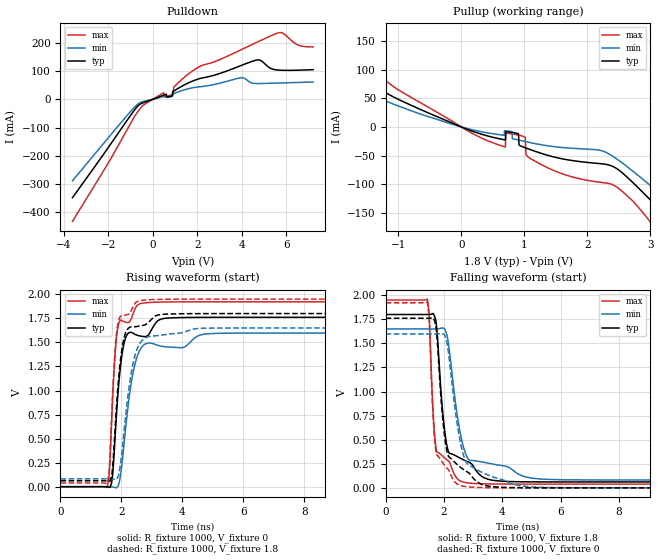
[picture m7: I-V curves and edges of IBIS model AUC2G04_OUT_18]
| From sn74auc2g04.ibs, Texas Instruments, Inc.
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[Model]   AUC2G04_OUT_18
Model_type  Output
Vref =   0
Rref =   1000
Cref =   30p
Vmeas =   0.9
| variable   typ   min   max
C_comp   6.69pF   0.47pF   21.38pF
| C_pullup   7.14pF   1.04pF   21.38pF
| C_pulldown   6.23pF   0.47pF   15.44pF
[Temperature Range]   40   100   -40
| Ambient temperature   25   85   -40
[Voltage range]   1.8   1.65   1.95
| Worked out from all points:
|   slope of the pulldown table from 0 to 0.27 V, typ, clamps not added: 34.4 ohm
|   slope of the pullup table from 0 to 0.27 V, typ, clamps not added: 24.7 ohm
|   rising waveform, R_fixture 1000, V_fixture 0: 20-80 % time 275ps typ, 402ps min, 194ps max; typ from 0 V to 1.76 V
|   falling waveform, R_fixture 1000, V_fixture 1.8: 20-80 % time 322ps typ, 477ps min, 201ps max; typ from 1.8 V to 0.061 V
|   rising waveform, R_fixture 1000, V_fixture 1.8: 20-80 % time 271ps typ, 394ps min, 192ps max; typ from 0.061 V to 1.8 V
|   falling waveform, R_fixture 1000, V_fixture 0: 20-80 % time 328ps typ, 487ps min, 200ps max; typ from 1.76 V to 0 V
[Pulldown]
| AUC2G04_OUT_18
|   Voltage   I(typ)   I(min)   I(max)
-3.6V     -347.8mA   -288mA     -431.4mA
-830mV    -38.95mA   -28.96mA   -62.23mA
-405mV    -11.33mA   -7.446mA   -19.55mA
495mV     14.95mA    10.62mA    23.51mA
885mV     12.27mA    19.08mA    15.87mA
925mV     28.56mA    20.18mA    16.89mA
960mV     30.12mA    21.17mA    44.33mA
2.04V     71.79mA    43.96mA    113.2mA
3.92V     118.2mA    75.86mA    173.7mA
4.625V    138.4mA    55.98mA    200.1mA
5.58V     103.9mA    57.6mA     233.8mA
7.2V      105mA      61.31mA    185.3mA
[Pullup]
| AUC2G04_OUT_18
|   Voltage   I(typ)   I(min)   I(max)
-3.6V     266.7mA    220.8mA    317.6mA
-2.61V    173.8mA    138mA      219.2mA
-2.13V    131.2mA    101.7mA    171.3mA
110mV     -4.812mA   -3.244mA   -7.318mA
695mV     -22.64mA   -6.826mA   -34.84mA
705mV     -8.168mA   -6.941mA   -10.57mA
980mV     -34.9mA    -24.66mA   -16.5mA
1.11V     -40.21mA   -27.81mA   -56.13mA
2.25V     -64.62mA   -42.31mA   -97.29mA
3.1V      -138.7mA   -111.5mA   -179.7mA
3.925V    -231.6mA   -189mA     -291.1mA
7.2V      -598.3mA   -503.7mA   -721.4mA
[Ramp]
| AUC2G04_OUT_18
| variable   typ   min   max
dV/dt_r   1.06/2.77E-10   0.97/4.04E-10   1.16/1.95E-10
dV/dt_f   1.05/3.29E-10   0.95/4.81E-10   1.15/2.06E-10
R_load = 1000
[Rising Waveform]
| AUC2G04_OUT_18
R_fixture =   1000
C_fixture =   0
L_fixture =   0
V_fixture =   0
V_fixture_min = 0
V_fixture_max = 0
|   Time   V(typ)   V(min)   V(max)
0s        7.645nV    26.05nV    1.116nV
1.525ns   -1.349mV   623.3uV    -8.358mV
1.6ns     -6.002mV   554.4uV    134.8mV
1.695ns   75.26mV    -2.222mV   804.5mV
1.88ns    947.6mV    2.94mV     1.649V
2.14ns    1.551V     618.1mV    1.711V
2.365ns   1.598V     1.16V      1.783V
2.62ns    1.566V     1.43V      1.903V
3.74ns    1.756V     1.449V     1.921V
22.5ns    1.761V     1.597V     1.922V
[Falling Waveform]
| AUC2G04_OUT_18
R_fixture =   1000
C_fixture =   0
L_fixture =   0
V_fixture =   1.8
V_fixture_min = 1.65
V_fixture_max = 1.95
|   Time   V(typ)   V(min)   V(max)
0s        1.8V       1.65V      1.95V
1.43ns    1.8V       1.65V      1.958V
1.495ns   1.8V       1.65V      1.768V
1.635ns   1.807V     1.65V      744.8mV
1.74ns    1.689V     1.65V      391.5mV
1.945ns   819.4mV    1.659V     332.3mV
2.105ns   433mV      1.579V     289.8mV
2.67ns    291.2mV    421.7mV    59.62mV
5.38ns    61.75mV    90.15mV    38.81mV
22.5ns    61.07mV    81.21mV    38.69mV
[Rising Waveform]
| AUC2G04_OUT_18
R_fixture =   1000
C_fixture =   0
L_fixture =   0
V_fixture =   1.8
V_fixture_min = 1.65
V_fixture_max = 1.95
|   Time   V(typ)   V(min)   V(max)
0s        61.05mV    81.2mV     38.68mV
1.525ns   59.75mV    81.69mV    31mV
1.6ns     56.9mV     81.58mV    182.4mV
1.695ns   150.9mV    79.18mV    853.5mV
1.875ns   1.001V     96.8mV     1.68V
2.115ns   1.581V     668.5mV    1.782V
2.33ns    1.662V     1.199V     1.836V
2.57ns    1.669V     1.472V     1.931V
4.68ns    1.8V       1.647V     1.95V
22.5ns    1.8V       1.65V      1.95V
[Falling Waveform]
| AUC2G04_OUT_18
R_fixture =   1000
C_fixture =   0
L_fixture =   0
V_fixture =   0
V_fixture_min = 0
V_fixture_max = 0
|   Time   V(typ)   V(min)   V(max)
0s        1.761V     1.597V     1.922V
1.43ns    1.761V     1.597V     1.927V
1.495ns   1.761V     1.597V     1.727V
1.635ns   1.764V     1.597V     697.4mV
1.73ns    1.662V     1.597V     366.1mV
2.08ns    412.8mV    1.531V     213mV
2.585ns   209.2mV    440.2mV    22.72mV
3.015ns   97.28mV    208.5mV    6.386mV
4.94ns    1.077mV    10.96mV    195.1uV
22.5ns    24.01uV    3.303uV    10.68uV
